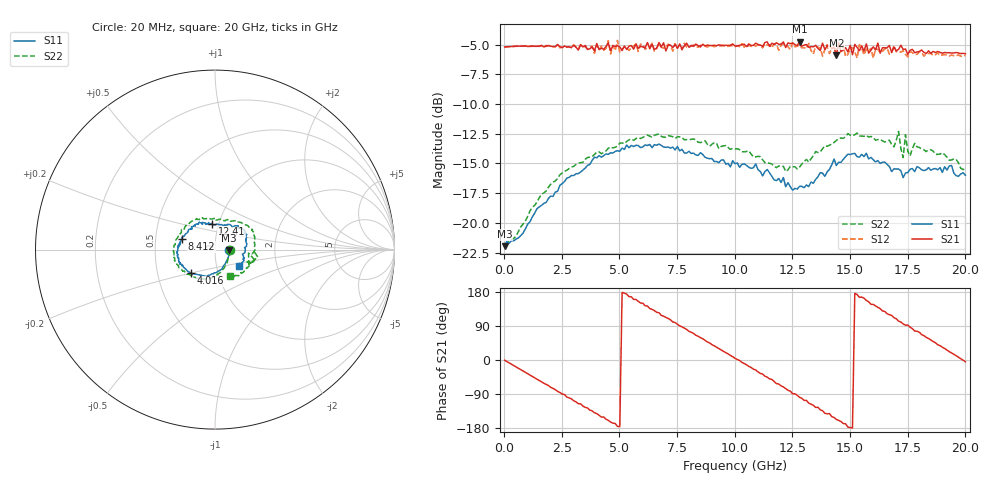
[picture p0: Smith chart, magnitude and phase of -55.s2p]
!Agilent Technologies,N5230A,US43500223,A.07.50.48
!Agilent N5230A: A.07.50.48
!Date: Saturday, September 19, 2015 14:44:31
!Correction: S11(Full 2 Port(1,2))
!S21(Full 2 Port(1,2))
!S12(Full 2 Port(1,2))
!S22(Full 2 Port(1,2))
!S2P File: Measurements: S11, S21, S12, S22:
# Hz S  RI  R 50
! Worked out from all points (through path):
!   201 points, 20 MHz to 20 GHz, reference 50 ohm
!   highest |S21| = -4.76 dB at 12.81 GHz (marker M1); lowest = -5.9 dB at 14.41 GHz (marker M2)
!   group delay of S21, straight-line fit = 100 ps
!   lowest |S11| = -22.0 dB at 20 MHz (marker M3), VSWR 1.17, Z = 58.7 - j0.351 ohm
!   |S11| at or under -10 dB: start of sweep to end of sweep
!   |S22| runs from -21.8 to -12.3 dB; largest |S21 - S12| = 0.075
!   S11 on the Smith chart (normalised r, x): 20 MHz: 1.17, -0.01; 4.016 GHz: 0.74, -0.20; 8.412 GHz: 0.69, +0.08; 12.41 GHz: 0.93, +0.27; 20 GHz: 1.28, -0.23
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2e7  0.0797 -0.00297  0.5491 -0.00551  0.5486 -0.0081  0.0808 -0.00252
9.191e8  0.0591 -0.0734  0.4689 -0.2963  0.4677 -0.2977  0.0617 -0.0809
1.8182e9  0.0176 -0.1205  0.2395 -0.4988  0.2381 -0.5043  0.018 -0.1347
3.4166e9  -0.0887 -0.1413  -0.2876 -0.468  -0.3056 -0.4617  -0.0829 -0.1592
4.016e9  -0.1335 -0.1319  -0.4434 -0.3543  -0.4311 -0.3576  -0.1245 -0.1544
4.9151e9  -0.176 -0.0971  -0.5535 -0.0457  -0.5833 -0.0434  -0.1732 -0.1185
5.7143e9  -0.2014 -0.066  -0.53 0.1951  -0.5292 0.2018  -0.2096 -0.0849
6.7133e9  -0.214 -0.0132  -0.3268 0.4707  -0.3166 0.4713  -0.2338 -0.0339
7.8122e9  -0.195 0.026  0.056 0.5515  0.0673 0.565  -0.2217 0.0274
8.4116e9  -0.1828 0.059  0.2557 0.4936  0.2528 0.4863  -0.2073 0.0684
1.001e10  -0.1208 0.1299  0.5525 0.0437  0.5497 0.0319  -0.137 0.1516
1.09091e10  -0.0893 0.1526  0.5104 -0.2536  0.4892 -0.2597  -0.0762 0.1733
1.18082e10  -0.0441 0.144  0.2651 -0.5068  0.2546 -0.5016  -0.016 0.1699
1.24076e10  -0.0171 0.1408  0.0759 -0.5616  0.0569 -0.5328  0.0284 0.1704
1.28072e10  0.00928 0.142  -0.0858 -0.5715  -0.082 -0.5551  0.0579 0.1612
1.34066e10  0.0563 0.1355  -0.2702 -0.4784  -0.2597 -0.4426  0.1053 0.16
1.44056e10  0.1272 0.1191  -0.4664 -0.2003  -0.503 -0.1899  0.1749 0.137
1.55045e10  0.1696 0.0945  -0.5388 0.1337  -0.5185 0.1682  0.2177 0.0791
1.67033e10  0.1718 0.0153  -0.2743 0.4853  -0.2481 0.4481  0.2225 -0.00316
1.81019e10  0.1506 -0.0723  0.2089 0.4907  0.2127 0.4762  0.1784 -0.0996
1.92008e10  0.147 -0.0784  0.4653 0.23  0.4626 0.2103  0.1221 -0.1442
2e10  0.1315 -0.0886  0.5125 -0.0392  0.5033 -0.0487  0.0813 -0.1477
